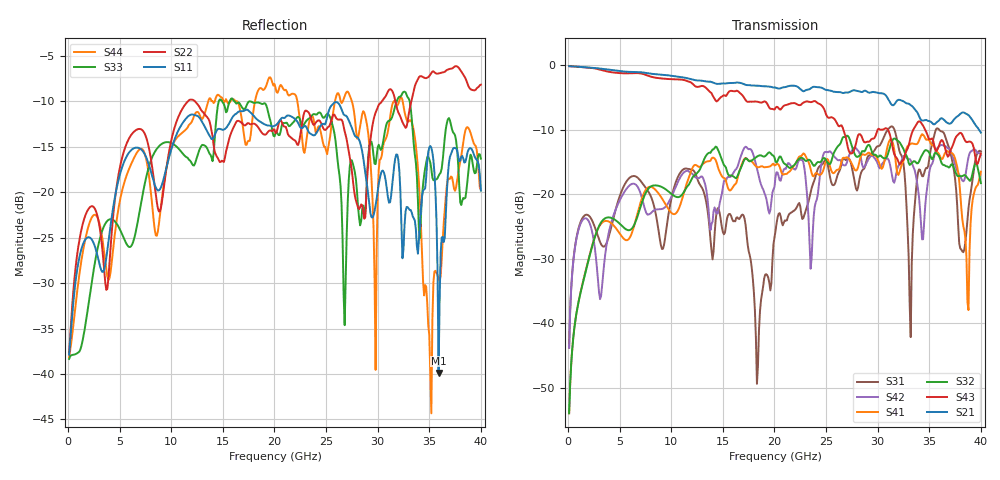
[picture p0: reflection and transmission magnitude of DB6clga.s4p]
! ADC12DJ3200QML-SP
! 196-pin ZMX package
! CLGA Ceramic Package without columns (ceramic land grid array)
! Texas Instruments 4/21/2021
! Single-ended  S-parameters
! PORT#  PORT_NAME  NET_NAME
! PORT1:  DAxN.DIEBUMP DAxN
! PORT2:  DAxN.BGA  DAxN
! PORT3:  DAxP.DIEBUMP DAxP
! PORT4:  DAxP.BGA  DAxP
! Touchstone Ver. 1.0
! Number of ports is 4
# Hz	S	MA	R	50.000000
! SCATTERING PARAMETERS  :
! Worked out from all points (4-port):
!   400 points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, 100 MHz to 40 GHz, reference 50 ohm
!   strongest paths, dB at 100 MHz, 10.1 GHz, 20.1 GHz, 30.1 GHz, 40 GHz:
!     S21: -0.1, -1.6, -3.4, -4.3, -10.4
!     S43: -0.1, -2.1, -6.6, -9.8, -13.7
!     S32: -54.0, -20.0, -14.9, -14.1, -18.3
!     S41: -54.0, -23.0, -15.5, -15.0, -16.5
!     S42: -43.8, -20.1, -17.3, -15.7, -13.9
!     S31: -43.8, -20.0, -25.7, -12.5, -13.4
!   lowest |S11| = -39.9 dB at 35.9 GHz (marker M1), VSWR 1.02, Z = 49.8 + j0.995 ohm
!   |S11| at or under -10 dB: start of sweep to end of sweep
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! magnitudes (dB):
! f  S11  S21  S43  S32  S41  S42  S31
! 100 MHz  -37.9  -0.1  -0.1  -54.0  -54.0  -43.8  -43.8
! 19.5 GHz  -12.7  -3.3  -6.6  -13.5  -15.7  -23.0  -33.7
! 29.8 GHz  -21.4  -4.2  -10.9  -13.9  -14.0  -14.6  -12.9
! 31.4 GHz  -19.3  -6.1  -12.3  -11.7  -11.7  -17.2  -9.5
! 33.2 GHz  -22.0  -6.2  -11.1  -15.3  -12.2  -14.7  -42.2
! 35.9 GHz  -39.9  -8.6  -12.6  -14.0  -13.6  -12.6  -9.9
! 40 GHz  -19.8  -10.4  -13.7  -18.3  -16.5  -13.9  -13.4
